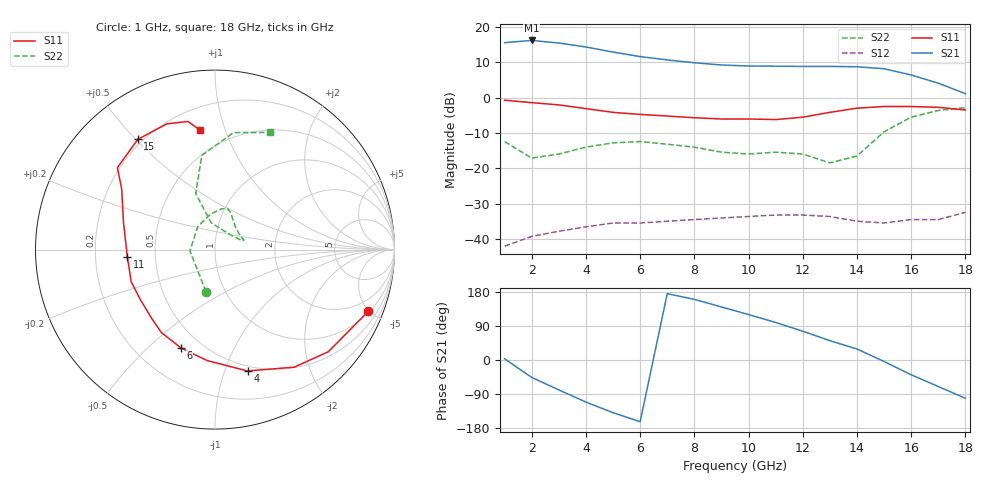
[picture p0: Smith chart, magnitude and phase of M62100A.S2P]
!  MGA-62100 S PARAMETERS
!  Vd=8V  Id=65mA  LAST UPDATED 07-22-92
# ghz s ma r 50
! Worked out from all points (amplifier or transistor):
!   18 points, 1 GHz to 18 GHz, reference 50 ohm
!   highest |S21| = 16.2 dB at 2 GHz (marker M1)
!   |S21| within 3 dB of that: start of sweep to 4.804 GHz
!   unconditionally stable (mu >= 1): start of sweep to end of sweep
!   at 4 GHz: K = 3.13, MAG = 17.5 dB, |S12| = -36.5 dB
!   at 10 GHz: K = 6.17, MAG = 10.4 dB, |S12| = -33.6 dB
!   at 18 GHz: K = 4.49, MAG = 7.3 dB, |S12| = -32.4 dB
!   S11 on the Smith chart (normalised r, x): 1 GHz: 1.09, -4.91; 4 GHz: 0.45, -1.20; 6 GHz: 0.39, -0.64; 11 GHz: 0.34, -0.04; 15 GHz: 0.18, +0.51; 18 GHz: 0.34, +0.82
1  0.92 -22.0  5.98 3.0  0.008 42.0  0.24 -102.0
2  0.85 -42.0  6.42 -46.0  0.011 50.0  0.14 -177.0
3  0.79 -56.0  5.91 -79.0  0.013 58.0  0.16 127.0
4  0.7 -75.0  5.19 -111.0  0.015 66.0  0.2 97.0
5  0.62 -94.0  4.4 -139.0  0.017 66.0  0.23 81.0
6  0.58 -109.0  3.8 -163.0  0.017 70.0  0.24 73.0
7  0.55 -123.0  3.41 175.0  0.018 75.0  0.22 66.0
8  0.52 -133.0  3.11 160.0  0.019 83.0  0.2 61.0
9  0.5 -147.0  2.89 140.0  0.02 85.0  0.17 48.0
10  0.5 -159.0  2.8 120.0  0.021 86.0  0.16 30.0
11  0.49 -175.0  2.78 99.0  0.022 81.0  0.17 18.0
12  0.53 164.0  2.76 76.0  0.022 70.0  0.16 18.0
13  0.62 147.0  2.76 51.0  0.021 49.0  0.12 42.0
14  0.71 140.0  2.73 29.0  0.018 21.0  0.15 98.0
15  0.75 125.0  2.56 -4.0  0.017 -27.0  0.33 109.0
16  0.75 111.0  2.09 -39.0  0.019 -76.0  0.53 98.0
17  0.73 102.0  1.6 -70.0  0.019 -119.0  0.66 81.0
18  0.67 97.0  1.14 -101.0  0.024 -137.0  0.72 65.0
